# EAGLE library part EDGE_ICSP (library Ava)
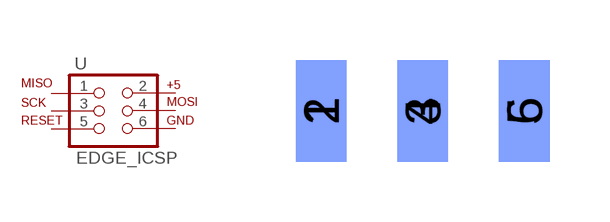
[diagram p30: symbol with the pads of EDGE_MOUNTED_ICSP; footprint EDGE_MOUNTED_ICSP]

Designator prefix -

## EDGE_ICSP  [EDGE_MOUNTED_ICSP]
1  1  pas
2  2  pas
3  3  pas
4  4  pas
5  5  pas
6  6  pas

## Footprint EDGE_MOUNTED_ICSP (pad centres in mm)
smd 1.27 x 2.54 bottom: 1 -2.54,0; 3 0,0; 5 2.54,0
smd 1.27 x 2.54: 2 -2.54,0; 4 0,0; 6 2.54,0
